(* Logix 5000 Routine export CANopenRouterB; software revision 24.00 *)

TYPE AparianString16 :   // string type
STRUCT
   LEN : DINT;
   DATA : SINT[16];
END_STRUCT
END_TYPE

TYPE AparianCANORBPassThroughRes :
STRUCT
   Status : INT;
   DataLength : INT;
   Data : SINT[480];
END_STRUCT
END_TYPE

TYPE AparianCANORBNodeOutput :
STRUCT
   SlaveDevTPDOTrig : BOOL[32];
END_STRUCT
END_TYPE

TYPE AparianCANORBNodeInput :
STRUCT
   SlaveAddr : SINT;
   Reserved0 : SINT;
   Online : BOOL;
   ErrRecv : BOOL;
   PDOErr : BOOL;
   Initalizing : BOOL;
   Stopped : BOOL;
   Operational : BOOL;
   PreOperational : BOOL;
   Reserved1 : BOOL;
   PDOMapOk : BOOL;
END_STRUCT
END_TYPE

TYPE AparianCANORBInputMap :
STRUCT
   CANData : SINT[500];
END_STRUCT
END_TYPE

TYPE AparianCANORBOutput02 :
STRUCT
   SlaveDevTPDOOutputTrig : AparianCANORBNodeOutput[124];
END_STRUCT
END_TYPE

TYPE AparianCANORBGenOp :
STRUCT
   NetPreOp : BOOL;
   NetStop : BOOL;
   Inhibit : BOOL;
END_STRUCT
END_TYPE

TYPE AparianCANORBOutput01 :
STRUCT
   GenOp : AparianCANORBGenOp;
   UTC : DINT[2];
   SlaveModeTPDOOutputTrig : BOOL[128];
END_STRUCT
END_TYPE

TYPE AparianCANORBInput01 :
STRUCT
   InstName : AparianString16;
   Status : AparianCANORBStatus;
   TransactionRate : DINT;
   Temperature : REAL;
   UTCTime : DINT[2];
   RxCanCount : DINT;
   TxCanCount : DINT;
   CanCrcErrCount : DINT;
   CanBitErrCount : DINT;
   CanStuffErrCount : DINT;
   CanBusOffCount : DINT;
   CanAckErrCount : DINT;
   CanFormatErrCount : DINT;
   PDOTxCount : DINT;
   PDORxCount : DINT;
   SDOTxCount : DINT;
   SDORxCount : DINT;
   TimePcktCount : DINT;
   SyncPcktCount : DINT;
   EmergencyPcktCount : DINT;
   HeartbeatPcktCount : DINT;
   TagReadCount : DINT;
   TagWriteCount : DINT;
   TagConnFailCount : DINT;
   TagErrCount : DINT;
END_STRUCT
END_TYPE

TYPE AparianCANORBPassThroughReq :
STRUCT
   Node : SINT;
   Function : SINT;
   Index : INT;
   SubIndex : INT;
   Reserved : INT;
   TimeoutTime : INT;
   DataLength : INT;
   Data : SINT[480];
END_STRUCT
END_TYPE

TYPE AparianCANORBOutputMap :
STRUCT
   CANData : SINT[500];
END_STRUCT
END_TYPE

TYPE AparianCANORBInput02 :
STRUCT
   Slaves : AparianCANORBNodeInput[124];
END_STRUCT
END_TYPE

TYPE AparianCANORBStatus :
STRUCT
   ConfigValid : BOOL;
   DupNode : BOOL;
   NetworkOperational : BOOL;
   NetworkPreOperational : BOOL;
   NetworkStopped : BOOL;
   MasterMode : BOOL;
   SlaveMode : BOOL;
   MBCommsOk : BOOL;
   CANCommsInhibit : BOOL;
   BottomPwr : BOOL;
   FrontPwr : BOOL;
   EIPCommsOk : BOOL;
END_STRUCT
END_TYPE

VAR_GLOBAL   (* controller tags *)
   CANORBInputDataMap02 : AparianCANORBInputMap;
   SdoMsgTrig : BOOL;
   CANORBOutputDataMap01 : AparianCANORBOutputMap;
   CANORBInputDataMap01 : AparianCANORBInputMap;
   CANORB_PtRes : AparianCANORBPassThroughRes;
   CANORBInput01 : AparianCANORBInput01 := (InstName := 'Master', Status.ConfigValid := 1, Status.NetworkOperational := 1, Status.MasterMode := 1, Status.FrontPwr := 1, TransactionRate := 18, Temperature := 30.862661, RxCanCount := 60, TxCanCount := 120, PDOTxCount := 329, PDORxCount := 213, SDOTxCount := 154, SDORxCount := 152, TimePcktCount := 30, SyncPcktCount := 59, EmergencyPcktCount := 31, HeartbeatPcktCount := 54, TagErrCount := 7189);
   CANORBOutput01 : AparianCANORBOutput01;
   CANORBOutput02 : AparianCANORBOutput02;
   CANORB_PtReq : AparianCANORBPassThroughReq;
   SdoMsg : MESSAGE;
        MessageParameters(MessageType := CIP Generic, RequestedLength := 400, ConnectedFlag := 2, ConnectionPath := CANORB, ServiceCode := 16#0070, ObjectType := 16#0417, TargetObject := 1, LocalElement := CANORB_PtReq, DestinationTag := CANORB_PtRes)
   CANORBOutputDataMap02 : AparianCANORBOutputMap;
   CANORBInput02 : AparianCANORBInput02;
END_VAR

PROGRAM MainProgram

ROUTINE CANopenRouterB   (* ladder *)
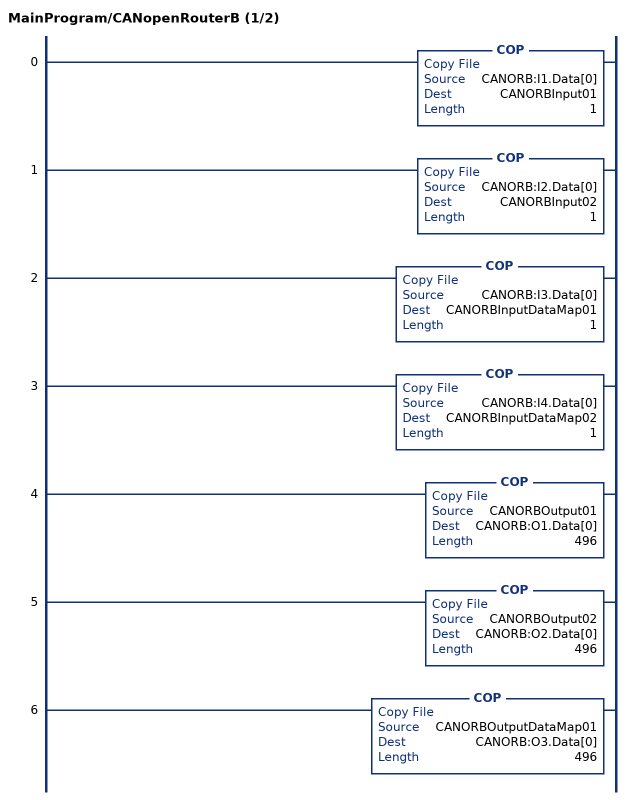
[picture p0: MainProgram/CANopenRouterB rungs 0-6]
   0: COP(CANORB:I1.Data[0],CANORBInput01,1);
   1: COP(CANORB:I2.Data[0],CANORBInput02,1);
   2: COP(CANORB:I3.Data[0],CANORBInputDataMap01,1);
   3: COP(CANORB:I4.Data[0],CANORBInputDataMap02,1);
   4: COP(CANORBOutput01,CANORB:O1.Data[0],496);
   5: COP(CANORBOutput02,CANORB:O2.Data[0],496);
   6: COP(CANORBOutputDataMap01,CANORB:O3.Data[0],496);
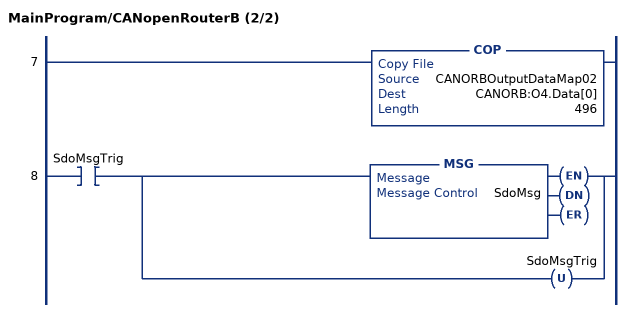
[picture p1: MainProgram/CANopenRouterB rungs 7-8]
   7: COP(CANORBOutputDataMap02,CANORB:O4.Data[0],496);
   8: XIC(SdoMsgTrig)[MSG(SdoMsg) ,OTU(SdoMsgTrig) ];
END_ROUTINE
END_PROGRAM
